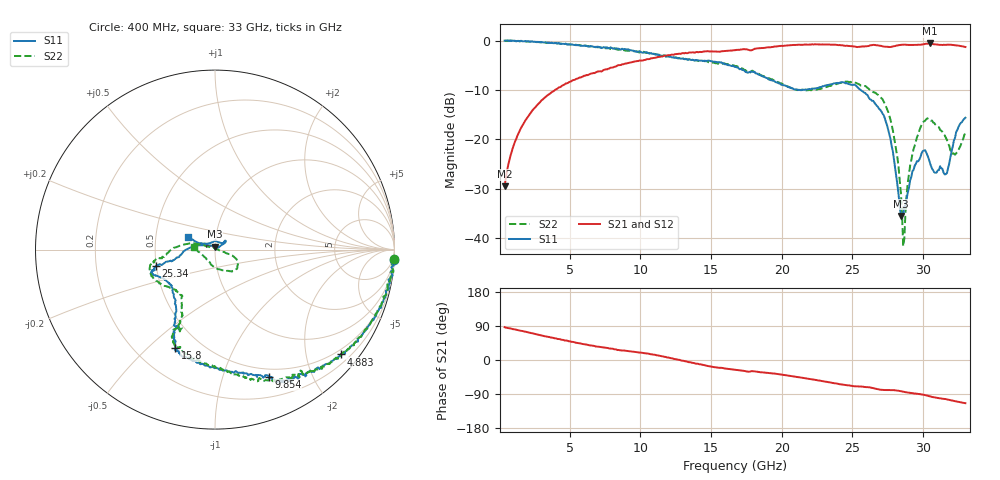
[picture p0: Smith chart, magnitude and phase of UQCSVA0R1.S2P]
!  Part Number  UQCSVA0R1  Mounting Orientation: Horizontal
!  Description: Ultra Low ESR Microwave capacitors
!  Application: Coupling, Bypass, Tuning, DC Block
!  Filters, Matching
# GHZ S DB R 50
! Freq  |S11|  S11 Ph  |S21|  S21 Ph  |S12|  S12 Ph  |S22|  S22 Ph
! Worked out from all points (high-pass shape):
!   401 points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, 400 MHz to 33 GHz, reference 50 ohm
!   highest |S21| = -0.57 dB at 30.47 GHz (marker M1); lowest = -29.5 dB at 400 MHz (marker M2)
!   |S21| within 3 dB of the highest: 10.87 GHz to end of sweep
!   lowest |S11| = -35.5 dB at 28.44 GHz (marker M3), VSWR 1.03, Z = 49.9 + j1.66 ohm
!   |S11| at or under -10 dB: 21.15567 GHz to 21.2478 GHz (92.13 MHz wide, 0.435 % of centre); 21.28 GHz to 21.46 GHz (181.1 MHz wide, 0.848 % of centre); 25.59 GHz to end of sweep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
!   |S22| runs from -41.7 to 0.0 dB; largest |S21 - S12| = 0.014
!   S11 on the Smith chart (normalised r, x): 400 MHz: 1, -34; 4.883 GHz: 0.39, -2.71; 9.854 GHz: 0.41, -1.43; 15.8 GHz: 0.36, -0.61; 25.34 GHz: 0.50, -0.10; 33 GHz: 0.73, +0.11
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0.4  -0.02 -3.4  -29.54 86.7  -29.54 86.4  -0.01 -3.0
1.949  -0.14 -15.8  -15.86 73.9  -15.89 73.7  -0.23 -15.6
4.883  -0.79 -39.8  -8.59 50.3  -8.57 49.5  -0.80 -39.6
5.861  -1.06 -46.7  -7.38 42.7  -7.40 42.5  -0.99 -46.6
9.854  -2.28 -67.2  -4.16 19.9  -4.17 19.6  -2.31 -70.5
11.321  -2.97 -75.8  -3.31 11.5  -3.39 11.0  -2.90 -78.7
15.804  -4.55 -111.9  -2.16 -21.0  -2.17 -21.4  -4.70 -110.2
16.7  -5.34 -114.8  -1.96 -25.5  -1.97 -25.9  -5.16 -115.4
22.161  -9.72 -149.0  -0.75 -51.0  -0.74 -51.0  -9.98 -133.8
25.339  -9.35 -164.6  -1.32 -69.7  -1.30 -69.7  -8.68 -167.0
27.051  -14.34 -171.4  -1.08 -78.5  -1.11 -78.7  -11.67 -176.3
27.621  -19.01 169.0  -1.31 -79.2  -1.29 -79.6  -15.28 170.4
28.11  -27.67 147.1  -1.02 -80.2  -1.02 -80.3  -22.36 161.4
28.436  -35.55 94.2  -0.87 -82.2  -0.86 -82.4  -30.80 154.2
28.681  -33.76 35.1  -0.82 -84.2  -0.83 -84.2  -40.16 19.0
29.007  -29.90 33.2  -0.89 -86.2  -0.90 -86.5  -27.14 -16.6
29.414  -25.37 34.1  -0.87 -88.5  -0.88 -88.3  -21.30 -17.2
30.066  -22.30 38.2  -0.75 -91.8  -0.75 -91.9  -16.36 -32.7
30.474  -24.63 36.6  -0.57 -95.8  -0.55 -95.8  -15.90 -47.4
31.615  -27.07 119.4  -0.88 -103.1  -0.86 -103.2  -19.66 -86.5
32.267  -19.73 157.9  -0.95 -108.7  -0.95 -108.9  -23.15 -138.0
33  -15.65 154.1  -1.31 -114.0  -1.30 -114.1  -18.74 173.6
